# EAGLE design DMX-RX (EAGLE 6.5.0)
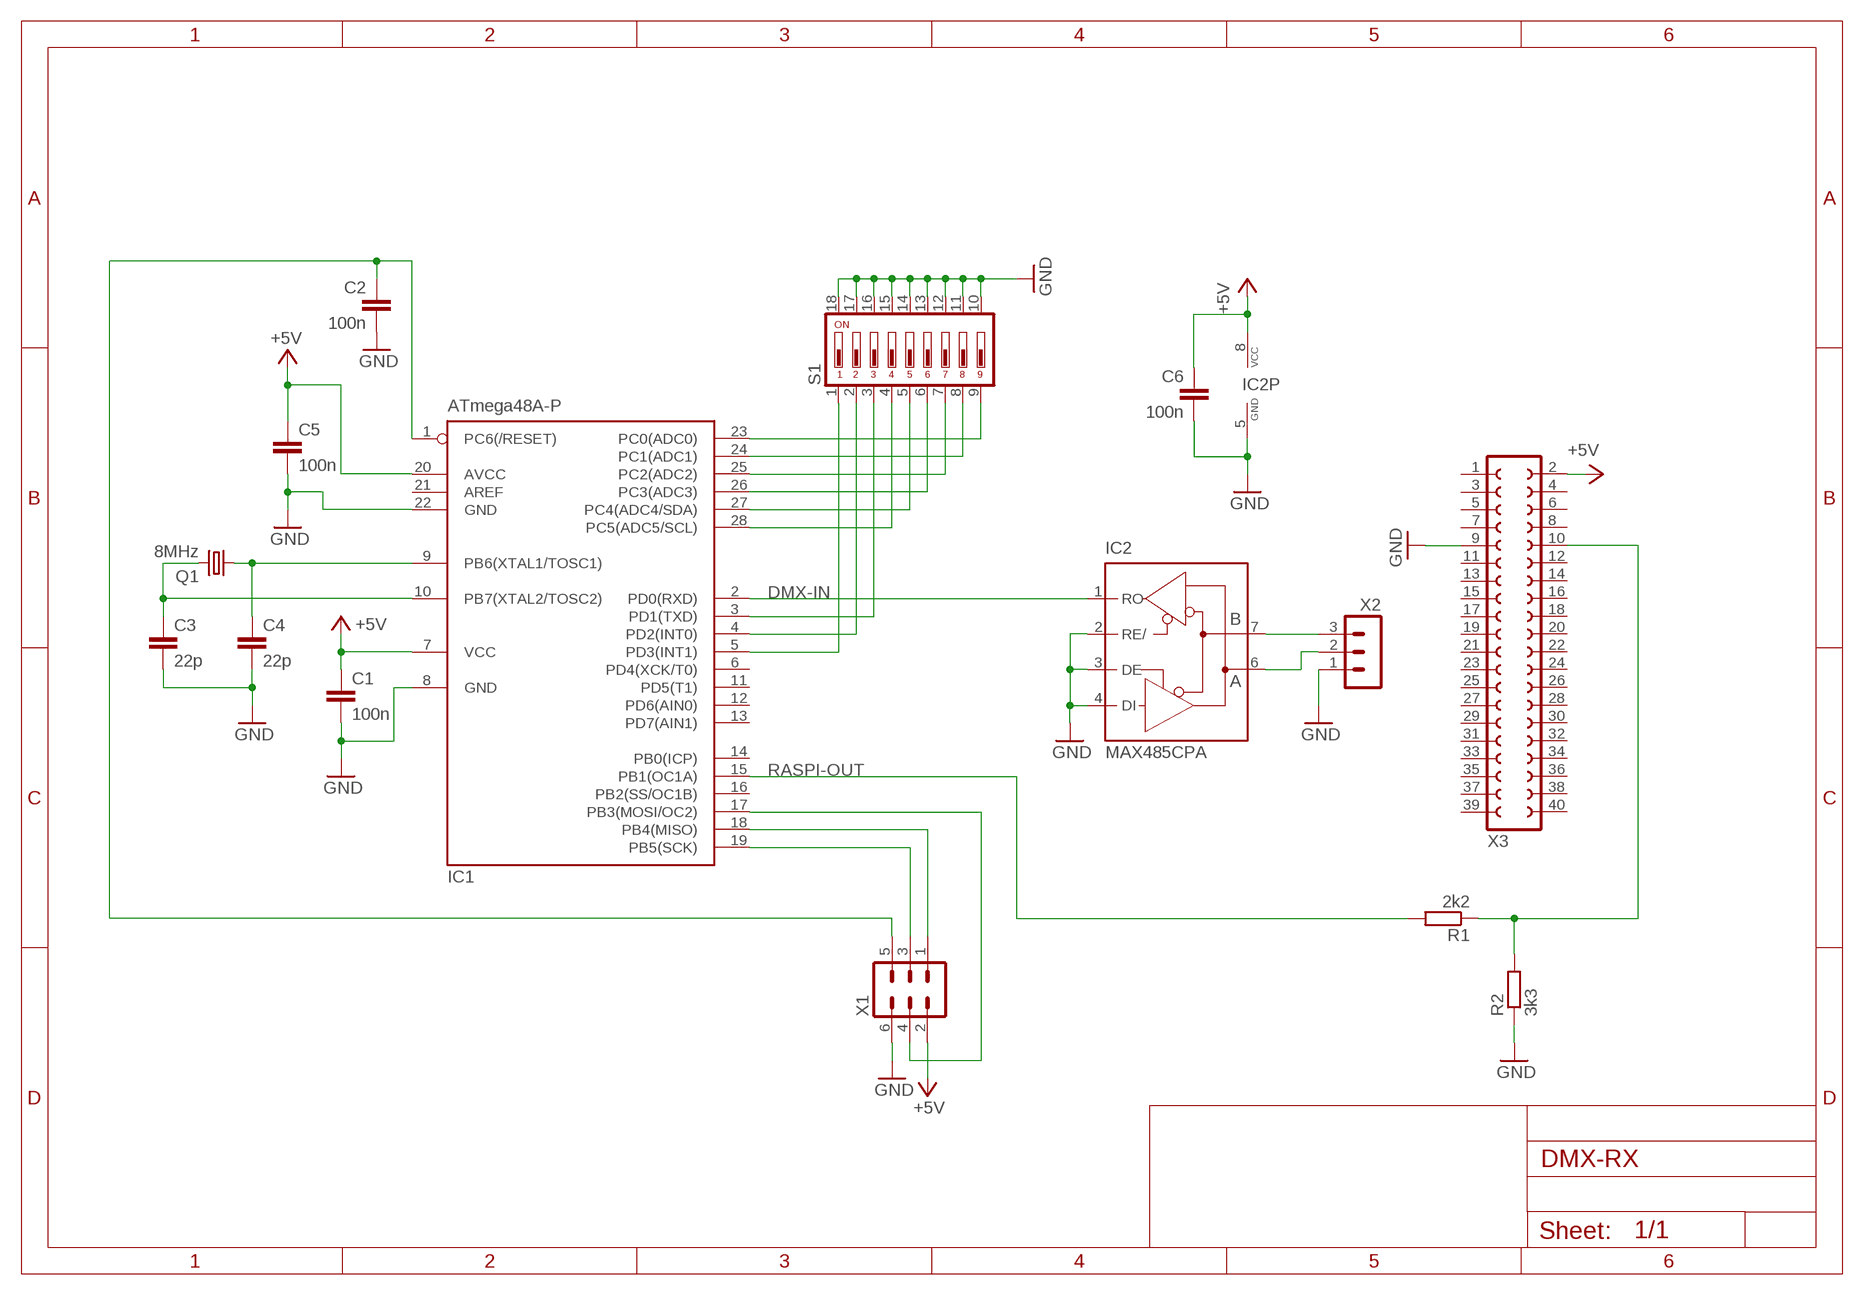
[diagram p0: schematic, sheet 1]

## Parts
C1  100n  C-EU025-024X044  [C025-024X044]
C2  100n  C-EU025-024X044  [C025-024X044]
C3  22p  C-EU025-024X044  [C025-024X044]
C4  22p  C-EU025-024X044  [C025-024X044]
C5  100n  C-EU025-024X044  [C025-024X044]
C6  100n  C-EU025-024X044  [C025-024X044]
IC1  ATmega48A-P  MEGA8-P  [DIL28-3]
IC2  MAX485CPA  MAX481CPA  [DIL08]
Q1  8MHz  CRYSTALHC49U-V  [HC49U-V]
R1  2k2  R-EU_0207/10  [0207/10]
R2  3k3  R-EU_0207/10  [0207/10]
S1  DIP09YL  [DIP09YL]
X1  ML6  [ML6]
X2  MA03-1  [MA03-1]
X3  FE20-2  [FE20-2]

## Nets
+5V: C1.1 C5.1 C6.1 IC1.7(VCC) IC1.20(AVCC) IC2.8(VCC) X1.2 X3.2
DMX-IN: IC1.2(PD0(RXD)) IC2.1(RO)
GND: C1.2 C2.2 C3.2 C4.2 C5.2 C6.2 IC1.8(GND) IC1.22(GND) IC2.2(RE/) IC2.3(DE) IC2.4(DI) IC2.5(GND) R2.1 S1.10 S1.11 S1.12 S1.13 S1.14 S1.15 S1.16 S1.17 S1.18 X1.6 X2.1 X3.9
N$1: C4.1 IC1.9(PB6(XTAL1/TOSC1)) Q1.1
N$2: C3.1 IC1.10(PB7(XTAL2/TOSC2)) Q1.2
N$3: IC2.7(B) X2.3
N$4: IC2.6(A) X2.2
N$6: C2.1 IC1.1(PC6(/RESET)) X1.5
N$9: IC1.18(PB4(MISO)) X1.1
N$10: IC1.5(PD3(INT1)) S1.1
N$11: IC1.4(PD2(INT0)) S1.2
N$12: IC1.3(PD1(TXD)) S1.3
N$13: IC1.28(PC5(ADC5/SCL)) S1.4
N$14: IC1.27(PC4(ADC4/SDA)) S1.5
N$15: IC1.26(PC3(ADC3)) S1.6
N$16: IC1.25(PC2(ADC2)) S1.7
N$17: IC1.24(PC1(ADC1)) S1.8
N$18: IC1.23(PC0(ADC0)) S1.9
N$20: IC1.19(PB5(SCK)) X1.3
N$22: IC1.17(PB3(MOSI/OC2)) X1.4
N$99: R1.1 R2.2 X3.10
RASPI-OUT: IC1.15(PB1(OC1A)) R1.2
Unconnected: IC1.6(PD4(XCK/T0)) IC1.11(PD5(T1)) IC1.12(PD6(AIN0)) IC1.13(PD7(AIN1)) IC1.14(PB0(ICP)) IC1.16(PB2(SS/OC1B)) IC1.21(AREF) X3.1 X3.3 X3.4 X3.5 X3.6 X3.7 X3.8 X3.11 X3.12 X3.13 X3.14 X3.15 X3.16 X3.17 X3.18 X3.19 X3.20 X3.21 X3.22 X3.23 X3.24 X3.25 X3.26 X3.27 X3.28 X3.29 X3.30 X3.31 X3.32 X3.33 X3.34 X3.35 X3.36 X3.37 X3.38 X3.39 X3.40

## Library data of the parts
C1-C6 = rcl:C-EU: CAPACITOR, European symbol
IC1 = atmel:MEGA8-P: MICROCONTROLLER 8 Kbytes FLASH, 1 kbytes SRAM, 512 bytes EEPROM, USART, 4-channel 10 bit ADC, 2-channel 8 bit ADC Pin compatible with Atmega48, ATMega88, ATMega168 Source: avr.lbr; OC_FARNELL: unknown; OC_NEWARK: unknown
IC2 = maxim:MAX481CPA: RS485 TRANSEIVER; MPN: MAX481CPA+; OC_FARNELL: unknown; OC_NEWARK: 99K3445
Q1 = crystal:CRYSTAL: CRYSTAL; OC_FARNELL: 1666969; OC_NEWARK: unknown
R1 R2 = rcl:R-EU_: RESISTOR, European symbol
S1 = switch-dil:DIP09YL: DIL/CODE SWITCH; OC_FARNELL: unknown; OC_NEWARK: unknown
X1 = con-harting-ml:ML6: HARTING; OC_FARNELL: unknown; OC_NEWARK: unknown
X2 = con-lstb:MA03-1: PIN HEADER; OC_FARNELL: unknown; OC_NEWARK: unknown
X3 = con-lsta:FE20-2: FEMALE HEADER; OC_FARNELL: unknown; OC_NEWARK: unknown

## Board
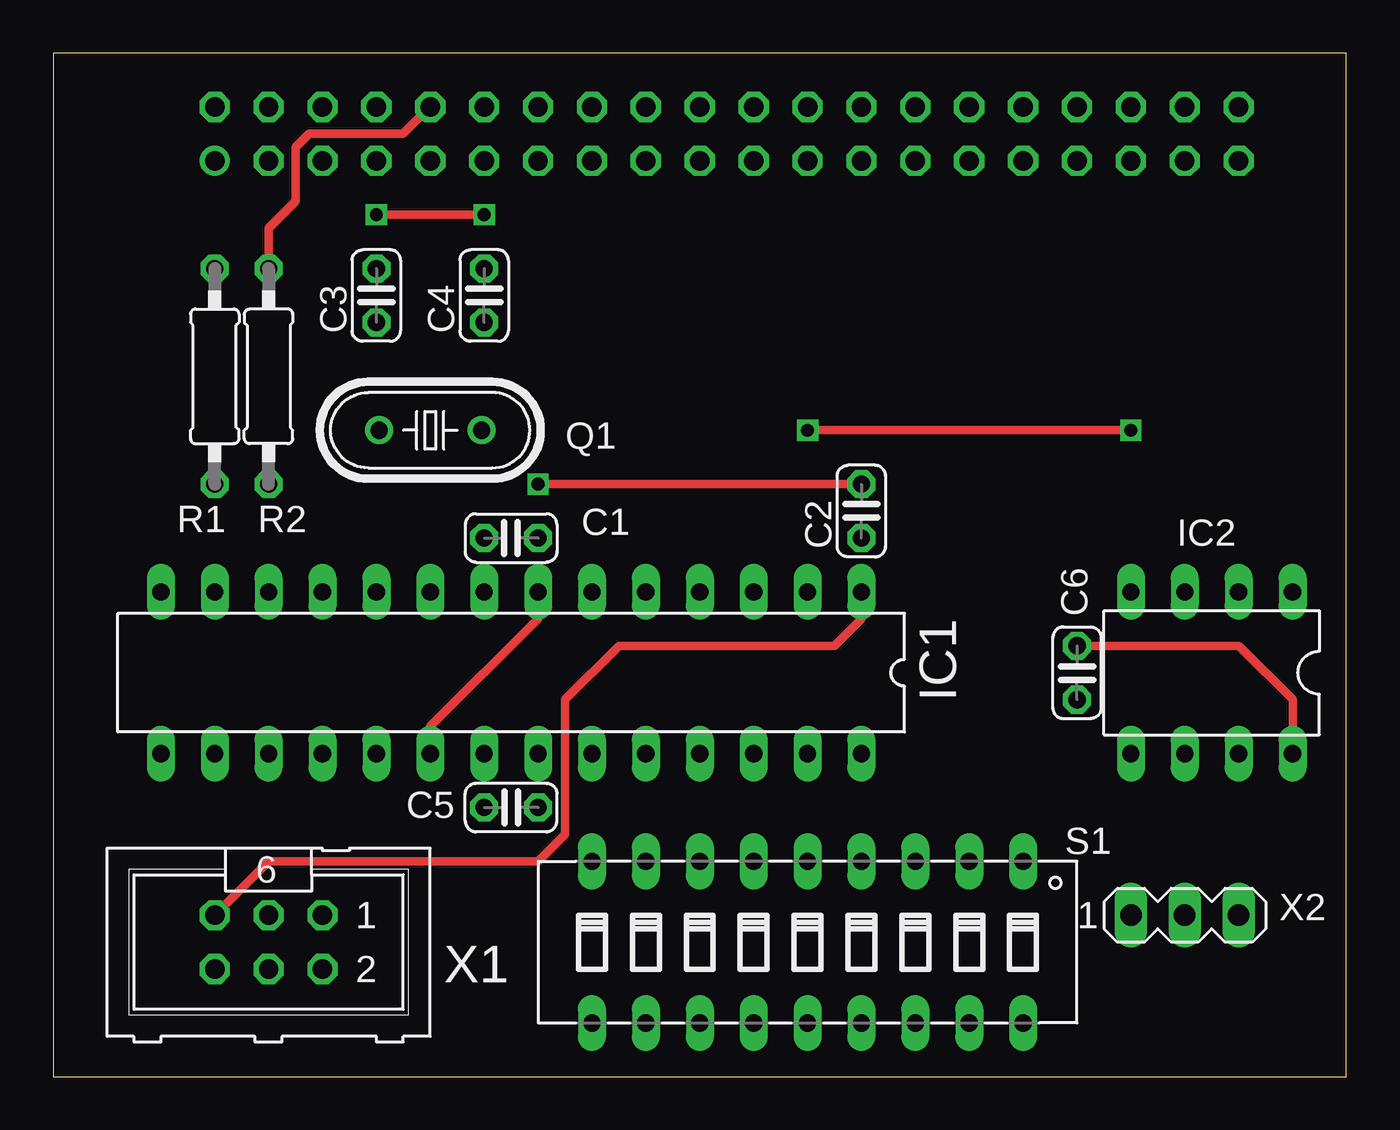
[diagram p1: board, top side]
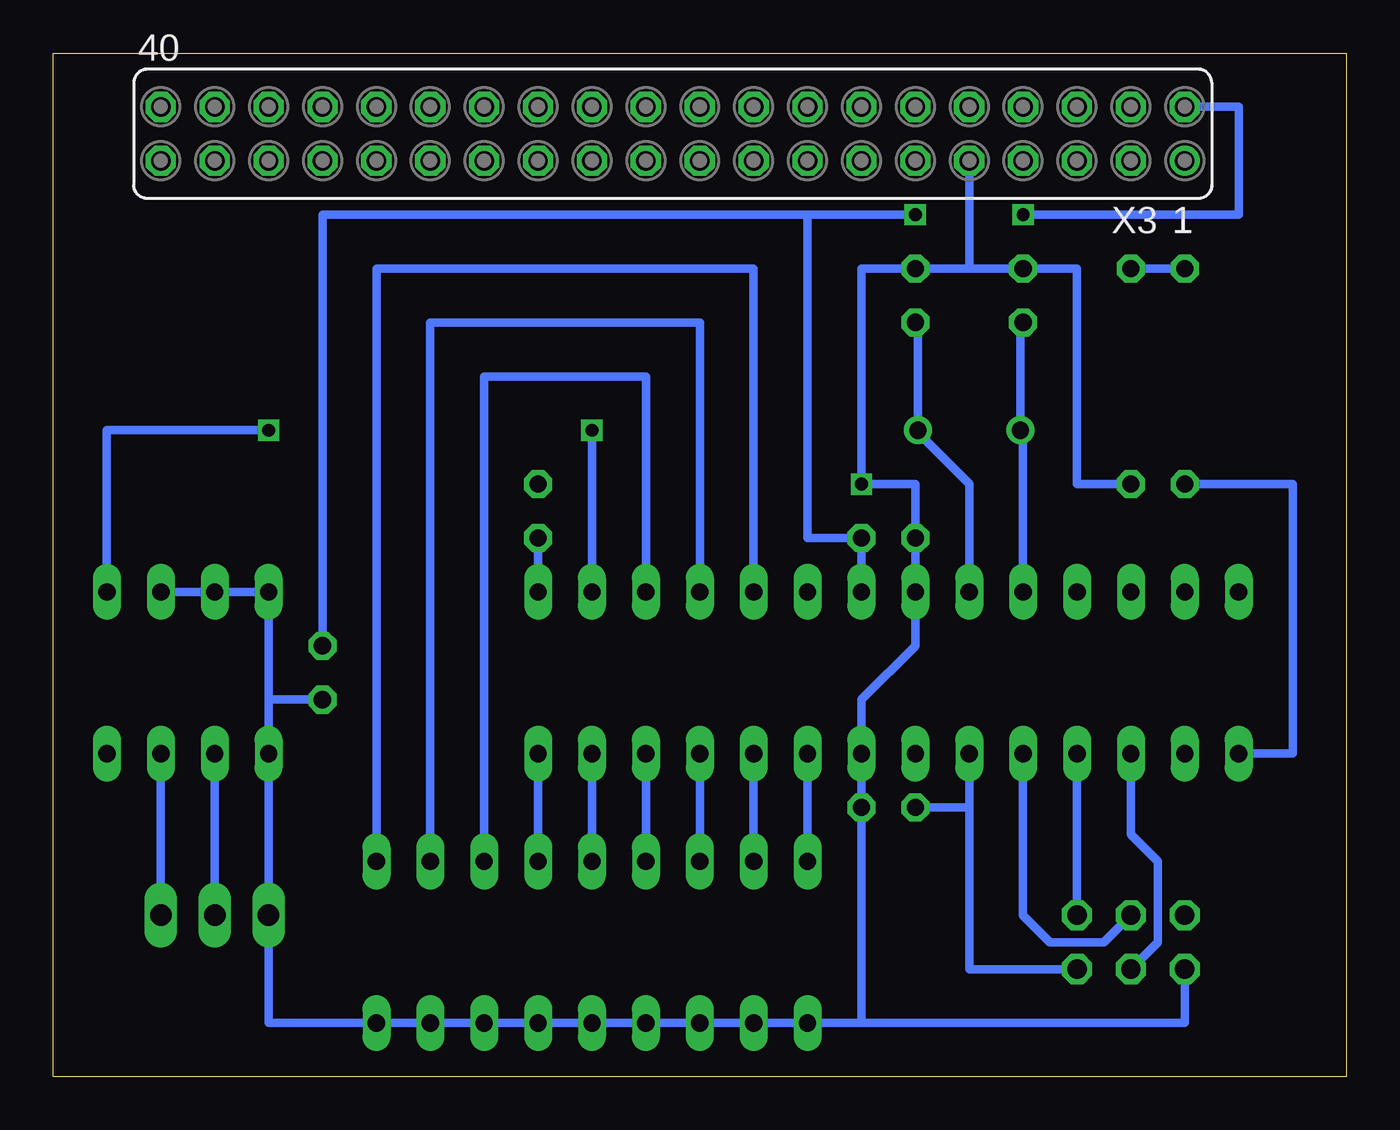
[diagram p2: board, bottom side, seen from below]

Size 60.96 x 48.26 mm. Coordinates in mm from the lower left corner, seen from the top.
Outline: 0,0 60.96,0 60.96,48.26 0,48.26 0,0
Copper layers (1*16): Top 0.035mm / dielectric 1.5mm / Bottom 0.035mm
Design rules "default *": minimum track width 10mil, minimum drill 0.6mm, track to track 8mil, track to pad 8mil, pad to pad 8mil, via to via 8mil, smd to smd 8mil, copper to edge 40mil, drill to drill 8mil, minimum pad ring 10mil, minimum via ring 8mil, stop-mask expansion 4mil, vias tented up to drill 0mil, thermal gap 10mil

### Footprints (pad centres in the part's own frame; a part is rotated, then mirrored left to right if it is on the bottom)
C025-024X044 = drill 0.813 octagon: 1 -1.27,0; 2 1.27,0
DIL28-3 = drill 0.813 long: 1 -16.51,-3.81; 2 -13.97,-3.81; 3 -11.43,-3.81; 4 -8.89,-3.81; 5 -6.35,-3.81; 6 -3.81,-3.81; 7 -1.27,-3.81; 8 1.27,-3.81; 9 3.81,-3.81; 10 6.35,-3.81; 11 8.89,-3.81; 12 11.43,-3.81; 13 13.97,-3.81; 14 16.51,-3.81; 15 16.51,3.81; 16 13.97,3.81; 17 11.43,3.81; 18 8.89,3.81; 19 6.35,3.81; 20 3.81,3.81; 21 1.27,3.81; 22 -1.27,3.81; 23 -3.81,3.81; 24 -6.35,3.81; 25 -8.89,3.81; 26 -11.43,3.81; 27 -13.97,3.81; 28 -16.51,3.81
DIL08 = drill 0.813 long: 1 -3.81,-3.81; 2 -1.27,-3.81; 3 1.27,-3.81; 4 3.81,-3.81; 5 3.81,3.81; 6 1.27,3.81; 7 -1.27,3.81; 8 -3.81,3.81
HC49U-V = drill 0.813: 1 -2.413,0; 2 2.413,0
0207/10 = drill 0.813 octagon: 1 -5.08,0; 2 5.08,0
DIP09YL = drill 0.813 long: 1 -10.16,-3.81; 2 -7.62,-3.81; 3 -5.08,-3.81; 4 -2.54,-3.81; 5 0,-3.81; 6 2.54,-3.81; 7 5.08,-3.81; 8 7.62,-3.81; 9 10.16,-3.81; 10 10.16,3.81; 11 7.62,3.81; 12 5.08,3.81; 13 2.54,3.81; 14 0,3.81; 15 -2.54,3.81; 16 -5.08,3.81; 17 -7.62,3.81; 18 -10.16,3.81
ML6 = drill 0.914 octagon: 1 -2.54,-1.27; 2 -2.54,1.27; 3 0,-1.27; 4 0,1.27; 5 2.54,-1.27; 6 2.54,1.27
MA03-1 = drill 1.016 long: 1 -2.54,0; 2 0,0; 3 2.54,0
FE20-2 = drill 0.914: 1 -24.13,1.27 | drill 0.914 octagon: 2 -24.13,-1.27; 3 -21.59,1.27; 4 -21.59,-1.27; 5 -19.05,1.27; 6 -19.05,-1.27; 7 -16.51,1.27; 8 -16.51,-1.27; 9 -13.97,1.27; 10 -13.97,-1.27; 11 -11.43,1.27; 12 -11.43,-1.27; 13 -8.89,1.27; 14 -8.89,-1.27; 15 -6.35,1.27; 16 -6.35,-1.27; 17 -3.81,1.27; 18 -3.81,-1.27; 19 -1.27,1.27; 20 -1.27,-1.27; 21 1.27,1.27; 22 1.27,-1.27; 23 3.81,1.27; 24 3.81,-1.27; 25 6.35,1.27; 26 6.35,-1.27; 27 8.89,1.27; 28 8.89,-1.27; 29 11.43,1.27; 30 11.43,-1.27; 31 13.97,1.27; 32 13.97,-1.27; 33 16.51,1.27; 34 16.51,-1.27; 35 19.05,1.27; 36 19.05,-1.27; 37 21.59,1.27; 38 21.59,-1.27; 39 24.13,1.27; 40 24.13,-1.27

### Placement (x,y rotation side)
C1  21.59,25.4 180 top
C2  38.1,26.67 90 top
C3  15.24,36.83 90 top
C4  20.32,36.83 90 top
C5  21.59,12.7 0 top
C6  48.26,19.05 270 top
IC1  21.59,19.05 180 top
IC2  54.61,19.05 180 top
Q1  17.78,30.48 180 top
R1  7.62,33.02 270 top
R2  10.16,33.02 90 top
S1  35.56,6.35 180 top
U$1  [A4L-LOC]  not placed on the board
X1  10.16,6.35 180 top
X2  53.34,7.62 0 top
X3  31.75,44.45 180 bottom

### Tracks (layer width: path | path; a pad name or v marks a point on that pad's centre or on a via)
+5V  (via drill 0.6)
  Top 0.406: C6.1 55.88,20.32 58.42,17.78 IC2.8 | v15.24,40.64 v20.32,40.64 | IC1.20 17.78,16.51 22.86,21.59 IC1.7
  Bottom 0.406: 17.78,12.7 IC1.20 | v15.24,40.64 5.08,40.64 5.08,45.72 X3.2 | IC1.7 C1.1 25.4,25.4 25.4,40.64 v20.32,40.64 48.26,40.64 C6.1 | X1.2 17.78,5.08 17.78,12.7 | 17.78,12.7 C5.1
DMX-IN  (via drill 0.6)
  Top 0.406: v35.56,30.48 v50.8,30.48
  Bottom 0.406: IC1.2 v35.56,30.48 | v50.8,30.48 58.42,30.48 IC2.1
GND  (via drill 0.6)
  Top 0.406: C2.2 v22.86,27.94
  Bottom 0.406: X3.9 17.78,38.1 C3.2 | C3.2 C4.2 22.86,38.1 v22.86,27.94 20.32,27.94 C1.2 IC1.8 20.32,20.32 22.86,17.78 IC1.22 C5.2 22.86,2.54 | 22.86,2.54 7.62,2.54 X1.6 | 50.8,17.78 IC2.5 X2.1 50.8,2.54 S1.18 S1.17 S1.16 S1.15 S1.14 S1.13 S1.12 S1.11 S1.10 22.86,2.54 | 50.8,17.78 C6.2 | IC2.2 IC2.3 IC2.4 50.8,17.78 | R2.1 12.7,27.94 12.7,38.1 C3.2
N$1
  Bottom 0.406: IC1.9 17.78,27.94 20.32,30.48 Q1.1 20.19,35.43 C4.1
N$2
  Bottom 0.406: IC1.10 15.24,30.35 Q1.2 15.37,35.43 C3.1
N$3
  Bottom 0.406: IC2.7 X2.3
N$4
  Bottom 0.406: X2.2 IC2.6
N$6
  Top 0.406: IC1.1 38.1,21.59 36.83,20.32 26.67,20.32 24.13,17.78 24.13,11.43 22.86,10.16 10.16,10.16 X1.5
  Bottom 0.406: C2.1 IC1.1
N$9
  Bottom 0.406: IC1.18 X1.1
N$10
  Bottom 0.406: S1.1 45.72,38.1 27.94,38.1 IC1.5
N$11
  Bottom 0.406: S1.2 43.18,35.56 30.48,35.56 IC1.4
N$12
  Bottom 0.406: S1.3 40.64,33.02 33.02,33.02 IC1.3
N$13
  Bottom 0.406: S1.4 IC1.28
N$14
  Bottom 0.406: IC1.27 S1.5
N$15
  Bottom 0.406: S1.6 IC1.26
N$16
  Bottom 0.406: IC1.25 S1.7
N$17
  Bottom 0.406: S1.8 IC1.24
N$18
  Bottom 0.406: IC1.23 S1.9
N$20
  Bottom 0.406: IC1.19 15.24,7.62 13.97,6.35 11.43,6.35 X1.3
N$22
  Bottom 0.406: IC1.17 10.16,11.43 8.89,10.16 8.89,6.35 X1.4
N$99
  Top 0.406: X3.10 16.51,44.45 12.06,44.45 11.43,43.81 11.43,41.27 10.16,40.01 R2.2
  Bottom 0.406: R2.2 R1.1
RASPI-OUT
  Bottom 0.406: IC1.15 2.54,15.24 2.54,27.94 R1.2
